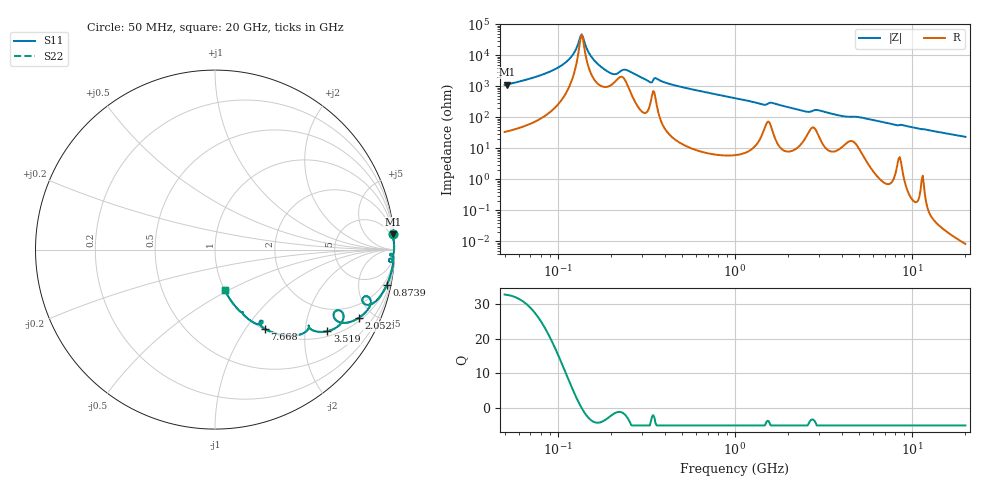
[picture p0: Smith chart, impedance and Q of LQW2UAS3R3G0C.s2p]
!Murata Part Number: LQW2UAS3R3G0C
!These Parameters are Measured in Series Mode Connection
!  o--[Z]--o
!Port1  Port2
!  o-------o
!Freq. Start=50[MHz] Stop=20[GHz], 401[Steps]
# Hz S RI R 50
!Freq.(Hz) S11(Real) S11(Imag) S21(Real) S21(Imag) S12(Real) S12(Imag) S22(Real) S22(Imag)
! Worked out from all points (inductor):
!   401 points, 50 MHz to 20 GHz, reference 50 ohm
!   read as one part in series: L = 3.02 uH near 51.52 MHz
!   highest Q = 32.6 at 51.52 MHz (marker M1), where L = 3.55 uH
!   self-resonance near 134.4 MHz
!   S11 on the Smith chart (normalised r, x): 50 MHz: 2, +22; 873.9 MHz: 1.12, -9.77; 2.052 GHz: 1.16, -4.12; 3.519 GHz: 1.16, -2.62; 7.668 GHz: 1.02, -1.23; 20 GHz: 1.00, -0.47
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5e7  0.9892 0.089  0.0108 -0.089  0.0108 -0.089  0.9892 0.089
5.152053e7  0.9899 0.0857  0.0101 -0.0857  0.0101 -0.0857  0.9899 0.0857
7.836543e7  0.9962 0.045  0.00379 -0.045  0.00379 -0.045  0.9962 0.045
1.026165e8  0.9979 0.0227  0.00212 -0.0227  0.00212 -0.0227  0.9979 0.0227
1.191979e8  0.9981 0.0108  0.00185 -0.0108  0.00185 -0.0108  0.9981 0.0108
1.323746e8  0.998 0.00236  0.002 -0.00236  0.002 -0.00236  0.998 0.00236
1.364002e8  0.9979 -8.25e-05  0.00211 8.25e-05  0.00211 8.25e-05  0.9979 -8.25e-05
1.560851e8  0.9968 -0.0115  0.00324 0.0115  0.00324 0.0115  0.9968 -0.0115
1.925012e8  0.9876 -0.0313  0.0124 0.0313  0.0124 0.0313  0.9876 -0.0313
2.106029e8  0.9762 -0.0314  0.0238 0.0314  0.0238 0.0314  0.9762 -0.0314
2.409965e8  0.9869 -0.0255  0.0131 0.0255  0.0131 0.0255  0.9869 -0.0255
3.300798e8  0.983 -0.0689  0.017 0.0689  0.017 0.0689  0.983 -0.0689
3.557498e8  0.9854 -0.0512  0.0146 0.0512  0.0146 0.0512  0.9854 -0.0512
3.721004e8  0.9915 -0.0615  0.00847 0.0615  0.00847 0.0615  0.9915 -0.0615
8.738837e8  0.9576 -0.1955  0.0424 0.1955  0.0424 0.1955  0.9576 -0.1955
1e9  0.9433 -0.2242  0.0567 0.2242  0.0567 0.2242  0.9433 -0.2242
2.05233e9  0.8 -0.3809  0.2 0.3809  0.2 0.3809  0.8 -0.3809
2.728004e9  0.6754 -0.3396  0.3246 0.3396  0.3246 0.3396  0.6754 -0.3396
3.519108e9  0.626 -0.4547  0.374 0.4547  0.374 0.4547  0.626 -0.4547
7.442007e9  0.2914 -0.4488  0.7086 0.4488  0.7086 0.4488  0.2914 -0.4488
7.668323e9  0.2768 -0.4409  0.7232 0.4409  0.7232 0.4409  0.2768 -0.4409
2e10  0.0531 -0.224  0.9469 0.224  0.9469 0.224  0.0531 -0.224
